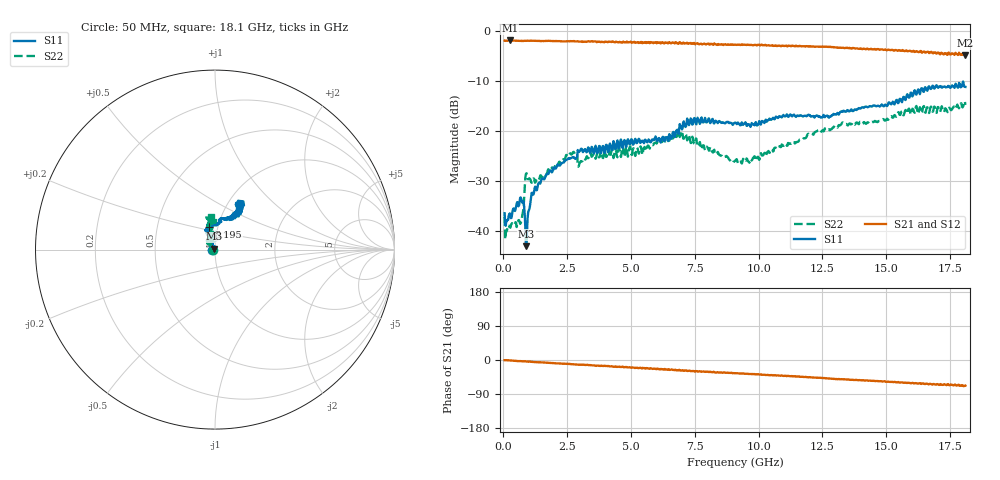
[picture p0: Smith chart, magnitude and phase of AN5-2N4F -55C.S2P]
! Network Analyzer HP8720D.06.14 Serial No. US36140669
! 12 Jan 2005  09:44:25
! Frequency  S11  S21  S12  S22
# HZ  S  DB R 50
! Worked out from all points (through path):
!   801 points, 50 MHz to 18.1 GHz, reference 50 ohm
!   highest |S21| = -1.91 dB at 253.1 MHz (marker M1); lowest = -4.9 dB at 18.1 GHz (marker M2)
!   group delay of S21, straight-line fit = 10.4 ps
!   lowest |S11| = -43.1 dB at 907.4 MHz (marker M3), VSWR 1.01, Z = 49.5 + j0.47 ohm
!   |S11| at or under -10 dB: start of sweep to end of sweep
!   |S22| runs from -41.7 to -14.1 dB; largest |S21 - S12| = 0.029
!   S11 on the Smith chart (normalised r, x): 50 MHz: 0.97, -0.01; 8.195 GHz: 0.90, +0.23; 18.1 GHz: 1.14, +0.59
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5e7  -36.51 -167.2  -1.94 -0.5  -1.98 -0.6  -37.26 -179.5
1.628125e8  -37.85 169.0  -1.97 -0.6  -1.97 -0.9  -39.34 179.9
2.530625e8  -36.54 160.0  -1.91 -1.1  -1.92 -1.5  -39.23 176.5
7.043125e8  -33.67 113.0  -1.98 -3.3  -1.99 -3.5  -38.08 -179.3
9.07375e8  -43.10 137.3  -1.98 -3.9  -1.98 -4.3  -28.49 164.3
9.525e8  -37.38 148.4  -1.96 -4.0  -1.95 -4.3  -29.62 153.6
1.04275e9  -35.05 140.3  -1.95 -4.3  -1.97 -4.8  -29.63 142.8
1.155562e9  -32.77 129.7  -2.00 -5.1  -1.99 -5.5  -29.68 140.4
1.448875e9  -30.55 120.3  -2.04 -6.2  -2.00 -6.5  -28.92 133.1
2.689812e9  -25.36 103.6  -2.05 -11.2  -2.07 -11.4  -24.68 120.8
3.073375e9  -23.63 98.4  -2.09 -12.7  -2.07 -12.8  -26.12 138.8
6.074188e9  -21.69 112.3  -2.35 -24.1  -2.35 -24.1  -22.41 116.8
6.931562e9  -18.92 109.3  -2.42 -28.1  -2.46 -27.4  -21.00 94.3
7.427938e9  -18.48 104.7  -2.56 -28.9  -2.56 -30.0  -21.73 72.7
8.195062e9  -17.61 105.4  -2.65 -32.5  -2.67 -32.1  -24.30 76.0
9.075e9  -18.38 114.1  -2.78 -34.6  -2.73 -35.0  -26.04 86.6
9.954938e9  -18.89 110.6  -2.82 -37.5  -2.79 -38.3  -25.25 94.7
1.103794e10  -17.13 106.0  -2.99 -41.6  -2.94 -42.4  -22.67 93.1
1.209838e10  -17.11 98.8  -3.12 -46.0  -3.10 -46.4  -20.55 102.2
1.509919e10  -14.30 68.8  -3.76 -57.5  -3.75 -57.5  -17.56 105.6
1.674625e10  -11.63 58.5  -4.22 -63.4  -4.21 -64.6  -15.16 91.6
1.81e10  -11.22 61.0  -4.90 -67.6  -4.90 -70.0  -14.82 97.9
